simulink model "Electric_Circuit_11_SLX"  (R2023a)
settings: Solver=ode23s  StartTime=0.0  StopTime=10.0  MaxStep=0.001  RelTol=1e-3
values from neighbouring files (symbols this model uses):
  C_3 = 0.001*F    (= 0.001)    [Electric_Circuit_11_EQN.m]    (also in Electric_Circuit_11_SLX_m.m; BIG_EC_Simscape_EQN.m; BIG_EC_Simscape_SLX_m.m; Electric_Circuit_03_EQN.m)
  C_7 = 0.001*F    (= 0.001)    [Electric_Circuit_11_EQN.m]    (also in Electric_Circuit_11_SLX_m.m; Electric_Circuit_02_EQN.m; Electric_Circuit_02_SLX_m.m; Electric_Circuit_04_EQN.m)
  C_8 = 0.001*F    (= 0.001)    [Electric_Circuit_11_EQN.m]    (also in Electric_Circuit_11_SLX_m.m; BIG_EC_Simscape_EQN.m; BIG_EC_Simscape_SLX_m.m; Hydraulic_Circuit_03_EQN.m)
  I_2_0 = 0*A    (= 0)    [Electric_Circuit_11_SLX_m.m]    (also in Electric_Circuit_02_SLX_m.m; Electric_Circuit_03_SLX_m.m; Electric_Circuit_06_SLX_m.m; Electric_Circuit_08_SLX_m.m)
  I_4_0 = 0*A    (= 0)    [Electric_Circuit_11_SLX_m.m]    (also in Electric_Circuit_02_SLX_m.m; Electric_Circuit_03_SLX_m.m; Electric_Circuit_04_SLX_m.m; Electric_Circuit_05_SLX_m.m)
  I_5_0 = 0*A    (= 0)    [Electric_Circuit_11_SLX_m.m]    (also in BIG_EC_Simscape_SLX_m.m; Electric_Circuit_01_SLX_m.m; Electric_Circuit_06_SLX_m.m; Electric_Circuit_09_SLX_m.m)
  I_9_0 = 0*A    (= 0)    [Electric_Circuit_11_SLX_m.m]    (also in BIG_EC_Simscape_SLX_m.m; Electric_Circuit_10_SLX_m.m)
  I_c_0 = 0*A    (= 0)    [Electric_Circuit_11_SLX_m.m]
  L_2 = 0.002*H    (= 0.002)    [Electric_Circuit_11_EQN.m]    (also in Electric_Circuit_11_SLX_m.m; Electric_Circuit_02_EQN.m; Electric_Circuit_02_SLX_m.m; Electric_Circuit_03_EQN.m)
  L_5 = 0.002*H    (= 0.002)    [Electric_Circuit_11_EQN.m]    (also in Electric_Circuit_11_SLX_m.m; BIG_EC_Simscape_EQN.m; BIG_EC_Simscape_SLX_m.m; Electric_Circuit_01_EQN.m)
  L_9 = 0.002*H    (= 0.002)    [Electric_Circuit_11_EQN.m]    (also in Electric_Circuit_11_SLX_m.m; BIG_EC_Simscape_EQN.m; BIG_EC_Simscape_SLX_m.m)
  R_6 = 100*Ohm    (= 100)    [Electric_Circuit_11_EQN.m]    (also in Electric_Circuit_11_SLX_m.m; BIG_EC_Simscape_EQN.m; BIG_EC_Simscape_SLX_m.m; Electric_Circuit_02_EQN.m)
  R_b = 100*Ohm    (= 100)    [Electric_Circuit_11_EQN.m]    (also in Electric_Circuit_11_SLX_m.m)
  Ts = Tfin/Nr_Ts_Points    (= 0.00144005)    [Electric_Circuit_11_SLX_m.m]    (also in BIG_EC_Simscape_SLX_m.m = 0.0003; Car_Dumper_SLX_m.m = 0.0022779; Electric_Circuit_01_SLX_m.m = 0.005; Electric_Circuit_02_SLX_m.m = 0.000480145)
  V_1_0 = 10*V    (= 10)    [Electric_Circuit_11_SLX_m.m]    (also in BIG_EC_Simscape_SLX_m.m; Electric_Circuit_02_SLX_m.m; Electric_Circuit_03_SLX_m.m; Electric_Circuit_04_SLX_m.m)
  V_3_0 = 0*V    (= 0)    [Electric_Circuit_11_SLX_m.m]    (also in BIG_EC_Simscape_SLX_m.m; Electric_Circuit_03_SLX_m.m; Electric_Circuit_07_SLX_m.m; Electrical_Transformer_SLX_m.m)
  V_7_0 = 0*V    (= 0)    [Electric_Circuit_11_SLX_m.m]    (also in Electric_Circuit_02_SLX_m.m; Electric_Circuit_04_SLX_m.m; Electric_Circuit_05_SLX_m.m; Electric_Circuit_07_SLX_m.m)
  V_8_0 = 0*V    (= 0)    [Electric_Circuit_11_SLX_m.m]    (also in BIG_EC_Simscape_SLX_m.m; Electric_Circuit_03_SLX_m.m; Electric_Circuit_04_SLX_m.m; Electric_Circuit_09_SLX_m.m)

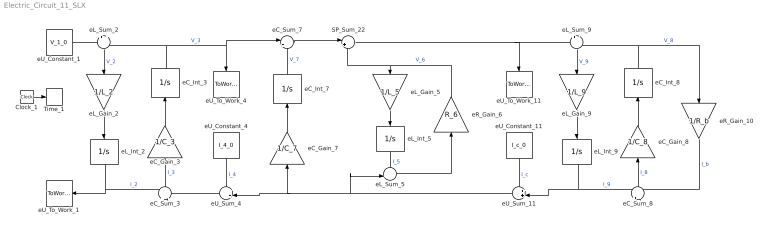
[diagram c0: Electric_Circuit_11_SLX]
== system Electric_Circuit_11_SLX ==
  Clock_1 : Clock
  SP_Sum_22 : Sum  Inputs=|+-
  Time_1 : ToWorkspace  VariableName=t  SaveFormat=Timeseries  SampleTime=Ts
  eC_Gain_3 : Gain  Gain=1/C_3  Multiplication=Matrix(K*u)
  eC_Gain_7 : Gain  Gain=1/C_7  Multiplication=Matrix(K*u)
  eC_Gain_8 : Gain  Gain=1/C_8  Multiplication=Matrix(K*u)
  eC_Int_3 : Integrator  InitialCondition=V_3_0
  eC_Int_7 : Integrator  InitialCondition=V_7_0
  eC_Int_8 : Integrator  InitialCondition=V_8_0
  eC_Sum_3 : Sum  Inputs=+|-
  eC_Sum_7 : Sum  Inputs=|+-
  eC_Sum_8 : Sum  Inputs=+|-
  eL_Gain_2 : Gain  Gain=1/L_2  Multiplication=Matrix(K*u)
  eL_Gain_5 : Gain  Gain=1/L_5  Multiplication=Matrix(K*u)
  eL_Gain_9 : Gain  Gain=1/L_9  Multiplication=Matrix(K*u)
  eL_Int_2 : Integrator  InitialCondition=I_2_0
  eL_Int_5 : Integrator  InitialCondition=I_5_0
  eL_Int_9 : Integrator  InitialCondition=I_9_0
  eL_Sum_2 : Sum  Inputs=+|-
  eL_Sum_5 : Sum  Inputs=-+|
  eL_Sum_9 : Sum  Inputs=+|-
  eR_Gain_10 : Gain  Gain=1/R_b  Multiplication=Matrix(K*u)
  eR_Gain_6 : Gain  Gain=R_6  Multiplication=Matrix(K*u)
  eU_Constant_1 : Constant  Value=V_1_0
  eU_Constant_11 : Constant  Value=I_c_0
  eU_Constant_4 : Constant  Value=I_4_0
  eU_Sum_11 : Sum  Inputs=++|
  eU_Sum_4 : Sum  Inputs=++|
  eU_To_Work_1 : ToWorkspace  VariableName=I_1_0  SaveFormat=Timeseries  SampleTime=Ts
  eU_To_Work_11 : ToWorkspace  VariableName=V_c_0  SaveFormat=Timeseries  SampleTime=Ts
  eU_To_Work_4 : ToWorkspace  VariableName=V_4_0  SaveFormat=Timeseries  SampleTime=Ts
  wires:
  eU_Constant_1/1 -> eL_Sum_2/1
  eC_Int_3/1 -> eL_Sum_2/2, eU_To_Work_4/1, eC_Sum_7/1  "V_3"
  eL_Int_2/1 -> eU_To_Work_1/1, eC_Sum_3/1  "I_2"
  eL_Sum_2/1 -> eL_Gain_2/1  "V_2"
  eL_Gain_2/1 -> eL_Int_2/1
  eU_Sum_4/1 -> eC_Sum_3/2
  eC_Sum_3/1 -> eC_Gain_3/1  "I_3"
  eC_Gain_3/1 -> eC_Int_3/1
  eU_Sum_11/1 -> eU_Sum_4/2, eC_Gain_7/1, eL_Sum_5/2
  eU_Constant_4/1 -> eU_Sum_4/1  "I_4"
  eC_Sum_7/1 -> SP_Sum_22/1
  eC_Gain_7/1 -> eC_Int_7/1
  eC_Int_7/1 -> eC_Sum_7/2  "V_7"
  SP_Sum_22/1 -> eU_To_Work_11/1, eL_Sum_9/1
  eR_Gain_6/1 -> SP_Sum_22/2, eL_Gain_5/1  "V_6"
  eL_Sum_5/1 -> eR_Gain_6/1
  eL_Gain_5/1 -> eL_Int_5/1
  eL_Int_5/1 -> eL_Sum_5/1  "I_5"
  eL_Int_9/1 -> eU_Sum_11/2, eC_Sum_8/1  "I_9"
  eU_Constant_11/1 -> eU_Sum_11/1  "I_c"
  eC_Int_8/1 -> eL_Sum_9/2, eR_Gain_10/1  "V_8"
  eL_Sum_9/1 -> eL_Gain_9/1  "V_9"
  eL_Gain_9/1 -> eL_Int_9/1
  eR_Gain_10/1 -> eC_Sum_8/2  "I_b"
  eC_Sum_8/1 -> eC_Gain_8/1  "I_8"
  eC_Gain_8/1 -> eC_Int_8/1
  Clock_1/1 -> Time_1/1
